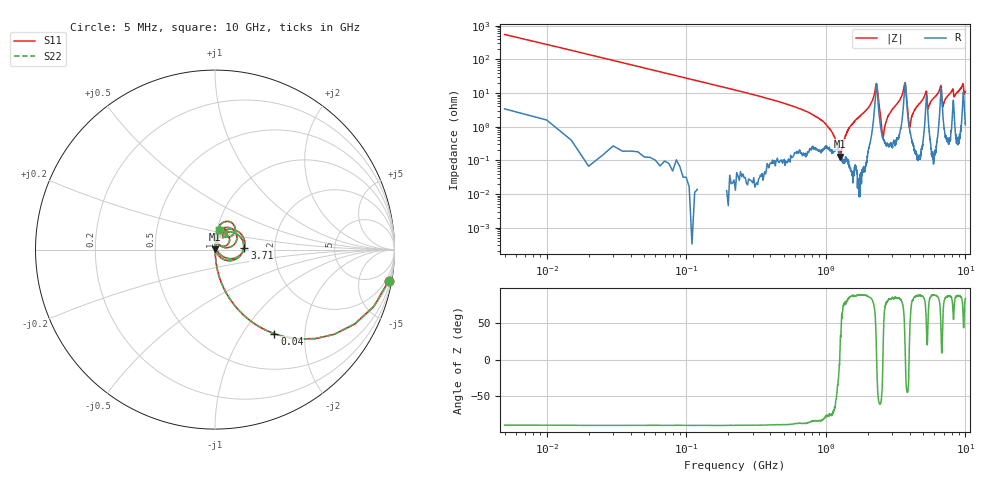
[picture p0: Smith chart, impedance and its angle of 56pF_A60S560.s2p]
! Amotech Co.,Ltd.
! http://www.amotech.co.kr/
! Part Number: A60S560
! These Parameters are Measured in Series Mode Connection
! Operation Temp=25[degC], DC Bias Voltage=0[V]
! Freq. Start=5[MHz] Stop=10[GHz], 2000[Steps]
! Date: Monday, July 13, 2020, 01:59:11
# GHZ S RI R 50.000000
!Freq.(Hz) S11(Real) S11(Imag) S21(Real) S21(Imag) S12(Real) S12(Imag) S22(Real) S22(Imag)
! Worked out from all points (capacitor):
!   2000 points, 5 MHz to 10 GHz, reference 50 ohm
!   read as one part in series: C = 56.4 pF near 55 MHz
!   lowest |Z| = 130 mohm at 1.27 GHz (marker M1)
!   series resonance near 1.258 GHz, so ESL is about 280 pH
!   S11 on the Smith chart (normalised r, x): 5 MHz: 1, -11; 40 MHz: 1.00, -1.41; 3.71 GHz: 1.39, +0.03; 10 GHz: 1.02, +0.22
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0.005  0.9673 -0.1749  0.0327 0.1749  0.0327 0.1749  0.9673 -0.1749
0.04  0.3313 -0.4693  0.6687 0.4693  0.6687 0.4693  0.3313 -0.4693
0.17  0.0263 -0.1602  0.9737 0.1602  0.9737 0.1602  0.0263 -0.1602
0.96  0.00241 -0.014  0.9976 0.014  0.9976 0.014  0.00241 -0.014
1.27  0.00116 0.000596  0.9988 -0.000596  0.9988 -0.000596  0.00116 0.000596
1.675  0.000809 0.0174  0.9992 -0.0174  0.9992 -0.0174  0.000809 0.0174
2.3  0.1544 0.0488  0.8456 -0.0488  0.8456 -0.0488  0.1544 0.0488
2.575  0.00428 0.00136  0.9957 -0.00136  0.9957 -0.00136  0.00428 0.00136
2.81  0.003 0.0215  0.997 -0.0215  0.997 -0.0215  0.003 0.0215
3.34  0.0084 0.0562  0.9916 -0.0562  0.9916 -0.0562  0.0084 0.0562
3.71  0.164 0.0098  0.836 -0.0098  0.836 -0.0098  0.164 0.0098
3.98  0.00865 0.00421  0.9914 -0.00421  0.9914 -0.00421  0.00865 0.00421
4.3  0.0031 0.0311  0.9969 -0.0311  0.9969 -0.0311  0.0031 0.0311
5.005  0.00943 0.0685  0.9906 -0.0685  0.9906 -0.0685  0.00943 0.0685
5.24  0.0691 0.0807  0.9309 -0.0807  0.9309 -0.0807  0.0691 0.0807
5.415  0.0176 0.0284  0.9824 -0.0284  0.9824 -0.0284  0.0176 0.0284
6.67  0.1115 0.1004  0.8885 -0.1004  0.8885 -0.1004  0.1115 0.1004
6.88  0.0252 0.0282  0.9748 -0.0282  0.9748 -0.0282  0.0252 0.0282
8.09  0.0432 0.1184  0.9568 -0.1184  0.9568 -0.1184  0.0432 0.1184
8.335  0.0232 0.073  0.9768 -0.073  0.9768 -0.073  0.0232 0.073
9.58  0.0824 0.1548  0.9176 -0.1548  0.9176 -0.1548  0.0824 0.1548
10  0.0233 0.1085  0.9767 -0.1085  0.9767 -0.1085  0.0233 0.1085
